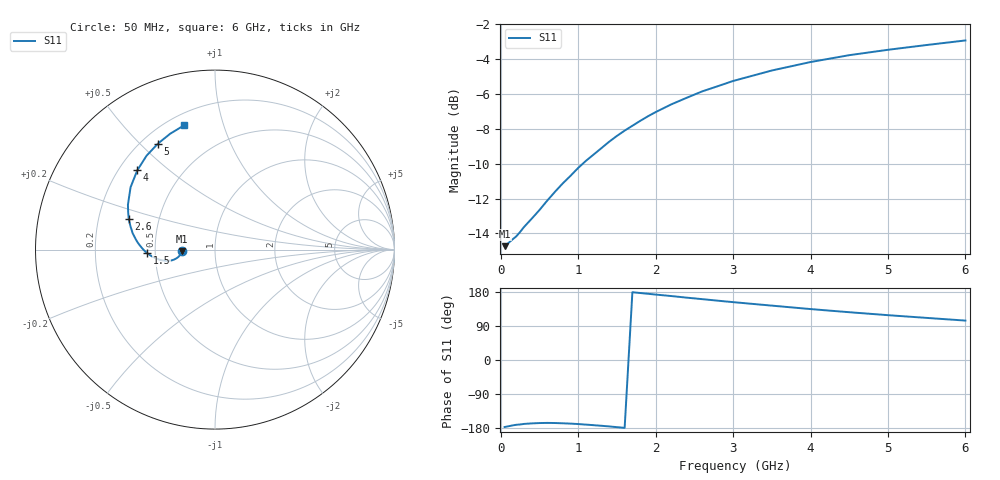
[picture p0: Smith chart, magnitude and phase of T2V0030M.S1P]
! SIEMENS Discrete & RF Semiconductors
! BAS70-04W
! Si Schottky Diode in SOT323
! IF = 30 mA
! S-Parameters:  November  1997
# GHz  S  MA  R  50
!  f  S11
! GHz  MAG  ANG
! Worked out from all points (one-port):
!   34 points, 50 MHz to 6 GHz, reference 50 ohm
!   lowest |S11| = -14.7 dB at 50 MHz (marker M1), VSWR 1.45, Z = 34.5 - j0.731 ohm
!   |S11| at or under -10 dB: start of sweep to 1.06 GHz
!   S11 on the Smith chart (normalised r, x): 50 MHz: 0.69, -0.01; 1.5 GHz: 0.45, -0.02; 2.6 GHz: 0.33, +0.15; 4 GHz: 0.27, +0.39; 5 GHz: 0.26, +0.57; 6 GHz: 0.26, +0.75
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0.05  0.1834 -176.8
0.2  0.1956 -171.0
0.25  0.2014 -170.1
0.3  0.2081 -168.7
0.4  0.2199 -167.3
0.5  0.2328 -166.4
0.6  0.2477 -166.0
0.7  0.2626 -166.3
0.8  0.2775 -167.0
1  0.3074 -169.0
1.1  0.3222 -170.5
1.3  0.3504 -173.6
1.4  0.3655 -175.3
1.5  0.3798 -177.2
1.6  0.3933 -179.1
1.8  0.4194 176.8
2  0.4445 172.7
2.2  0.4676 168.8
2.4  0.4885 164.6
2.6  0.5095 160.6
2.8  0.5272 156.6
3  0.5459 152.7
3.5  0.585 143.5
4  0.6187 134.4
4.5  0.6473 126.1
5  0.6707 118.3
5.5  0.6923 111.1
6  0.7134 104.0
